| Teraspeed Modeling Services.
| http://www.teraspeed.com
[IBIS Ver]   4.0
[Comment Char] |_char
[File Name]   lpc15xxjbd100.ibs
[File Rev]   3.0
[Source]  Measured and created by Teraspeed Consulting Group LLC
[Date]   03-05-2014
[Notes]   Quality Check of this IBIS model: Model Passes IBIS Check
   Model parses into ICX IS. Simulation done with Hyperlynx.
   1. MIN TYP MAX information is based on Temperature and Voltage
   characteristics only.
   2. Package data measured using Tektronix IConnect Software.
[Disclaimer]
| Use: Teraspeed Consulting Group LLC ("Teraspeed") has
| licensed IBIS models to specific integrated circuit
| suppliers ("IC Vendors") for use and distribution as
| follows: Each IC Vendor may use IBIS Models, and distribute
| them to IC Vendor's customers to use solely for developing
| printed circuit board designs. Users of this model may
| modify the IBIS model to suit its specific applications but
| rights to derivative works and such modifications shall belong
| to Teraspeed. No other distribution of these materials is
| permitted.
| DISCLAIMER OF WARRANTY: UNLESS OTHERWISE AGREED TO IN WRITING
| TERASPEED DISCLAIMS AND USER WAIVES ALL WARRANTIES, EXPRESS
| OR IMPLIED, INCLUDING WARRANTIES OF MERCHANTABILITY AND
| FITNESS FOR A PARTICULAR PURPOSE. IN NO EVENT SHALL
| TERASPEED BE LIABLE FOR ANY DIRECT OR INDIRECT DAMAGES,
| WHETHER IN CONTRACT OR TORT, INCLUDING, WITHOUT LIMITATION,
| LOST PROFITS, BUSINESS INTERRUPTION, OR LOST INFORMATION
| ARISING OUT OF THE USE OF OR THE INABILITY TO USE THE MODEL,
| EVEN IF TERASPEED HAS BEEN ADVISED OF THE POSSIBILITY OF SUCH
| DAMAGES.
[Copyright]
| This file is the legal property of Teraspeed Copyright(c) 2014.
| All other rights are reserved.
[Component]LPC15xxJBD100
[Manufacturer] NXP Semiconductors
[Package]
| variable   typ   min   max
| qfp100
R_pkg  1.917E-02   1.414E-02   2.417E-02
L_pkg  3.087E-09   2.277E-09   3.891E-09
C_pkg  6.299E-13   4.647E-13   7.940E-13
[Pin] signal_name  model_name  R_pin  L_pin C_pin
1   PIO0_30 pio0_30 2.417E-02   3.891E-09   7.940E-13
2   PIO0_0  pio0_0  2.326E-02   3.745E-09   7.642E-13
3   PIO0_31 pio0_31 2.236E-02   3.600E-09   7.347E-13
4   VDD   POWER   2.147E-02   3.457E-09   7.055E-13
5   PIO1_0  pio1_0  2.059E-02   3.315E-09   6.766E-13
6   PIO0_1  pio0_1  1.972E-02   3.175E-09   6.480E-13
7   VSS   GND   1.887E-02   3.038E-09   6.200E-13
8   PIO0_2  pio0_2  1.803E-02   2.903E-09   5.923E-13
9   PIO1_12 pio1_12 1.721E-02   2.770E-09   5.653E-13
10   PIO0_3  pio0_3  1.640E-02   2.641E-09   5.389E-13
11   PIO1_13 pio1_13 1.562E-02   2.515E-09   5.132E-13
12   PIO1_14 pio1_14 1.487E-02   2.393E-09   4.885E-13
13   PIO0_4  pio0_4  1.414E-02   2.277E-09   4.647E-13
14   PIO0_5  pio0_5  1.487E-02   2.393E-09   4.885E-13
15   PIO1_15 pio1_15 1.562E-02   2.515E-09   5.132E-13
16   PIO0_6  pio0_6  1.640E-02   2.641E-09   5.389E-13
17   PIO0_7  pio0_7  1.721E-02   2.770E-09   5.653E-13
18   PIO1_16 pio1_16 1.803E-02   2.903E-09   5.923E-13
19   PIO0_8  pio0_8  1.887E-02   3.038E-09   6.200E-13
20   PIO1_17 pio1_17 1.972E-02   3.175E-09   6.480E-13
21   VREFP_ADC POWER 2.059E-02   3.315E-09   6.766E-13
22   VREFN   POWER   2.147E-02   3.457E-09   7.055E-13
23   PIO1_1  pio1_1  2.236E-02   3.600E-09   7.347E-13
24   PIO0_9  pio0_9  2.326E-02   3.745E-09   7.642E-13
25   PIO1_18 pio1_18 2.417E-02   3.891E-09   7.940E-13
26   PIO0_18 pio0_18 2.417E-02   3.891E-09   7.940E-13
27   VREFP_DAC_VDDCMP POWER  2.326E-02   3.745E-09   7.642E-13
28   PIO0_10 pio0_10 2.236E-02   3.600E-09   7.347E-13
29   PIO1_19 pio1_19 2.147E-02   3.457E-09   7.055E-13
30   VDDA   POWER   2.059E-02   3.315E-09   6.766E-13
31   VSSA   GND   1.972E-02   3.175E-09   6.480E-13
32   VDD   POWER   1.887E-02   3.038E-09   6.200E-13
33   PIO0_11 pio0_11 1.803E-02   2.903E-09   5.923E-13
34   PIO1_20 pio1_20 1.721E-02   2.770E-09   5.653E-13
35   PIO0_12 pio0_12 1.640E-02   2.641E-09   5.389E-13
36   PIO1_2  pio1_2  1.562E-02   2.515E-09   5.132E-13
37   PIO1_21 pio1_21 1.487E-02   2.393E-09   4.885E-13
38   PIO1_22 pio1_22 1.414E-02   2.277E-09   4.647E-13
39   VSS   GND   1.487E-02   2.393E-09   4.885E-13
40   VSS   GND   1.562E-02   2.515E-09   5.132E-13
41   PIO1_3  pio1_3  1.640E-02   2.641E-09   5.389E-13
42   PIO1_23 pio1_23 1.721E-02   2.770E-09   5.653E-13
43   PIO0_13 pio0_13 1.803E-02   2.903E-09   5.923E-13
44   PIO1_24 pio1_24 1.887E-02   3.038E-09   6.200E-13
45   PIO0_14 pio0_14 1.972E-02   3.175E-09   6.480E-13
46   PIO1_25 pio1_25 2.059E-02   3.315E-09   6.766E-13
47   PIO0_15 pio0_15 2.147E-02   3.457E-09   7.055E-13
48   PIO1_26 pio1_26 2.236E-02   3.600E-09   7.347E-13
49   PIO0_16 pio0_16 2.326E-02   3.745E-09   7.642E-13
50   PIO1_27 pio1_27 2.417E-02   3.891E-09   7.940E-13
51   PIO1_4  pio1_4  2.417E-02   3.891E-09   7.940E-13
52   PIO1_5  pio1_5  2.326E-02   3.745E-09   7.642E-13
53   XTALOUT term   2.236E-02   3.600E-09   7.347E-13
54   XTALIN  xtalin  2.147E-02   3.457E-09   7.055E-13
55   PIO1_28 pio1_28 2.059E-02   3.315E-09   6.766E-13
56   PIO1_29 pio1_29 1.972E-02   3.175E-09   6.480E-13
57   VDD   POWER   1.887E-02   3.038E-09   6.200E-13
58   PIO1_11 pio1_11 1.803E-02   2.903E-09   5.923E-13
59   PIO1_30 pio1_30 1.721E-02   2.770E-09   5.653E-13
60   PIO1_31 pio1_31 1.640E-02   2.641E-09   5.389E-13
61   PIO0_17 pio0_17 1.562E-02   2.515E-09   5.132E-13
62   PIO2_0  pio2_0  1.487E-02   2.393E-09   4.885E-13
63   PIO0_19 pio0_19 1.414E-02   2.277E-09   4.647E-13
64   PIO2_1  pio2_1  1.487E-02   2.393E-09   4.885E-13
65   VBAT   POWER   1.562E-02   2.515E-09   5.132E-13
66   RTCXIN  rtcxin  1.640E-02   2.641E-09   5.389E-13
67   RTCXOUT rtcxout 1.721E-02   2.770E-09   5.653E-13
68   VSS   GND   1.803E-02   2.903E-09   5.923E-13
69   PIO0_20 pio0_20 1.887E-02   3.038E-09   6.200E-13
70   VDD   POWER   1.972E-02   3.175E-09   6.480E-13
71   RESET   pio0_20 2.059E-02   3.315E-09   6.766E-13
72   PIO2_2  pio2_2  2.147E-02   3.457E-09   7.055E-13
73   PIO1_6  pio1_6  2.236E-02   3.600E-09   7.347E-13
74   PIO2_12 pio2_12 2.326E-02   3.745E-09   7.642E-13
75   PIO2_13 pio2_13 2.417E-02   3.891E-09   7.940E-13
76   PIO2_3  pio2_3  2.417E-02   3.891E-09   7.940E-13
77   PIO2_4  pio2_4  2.326E-02   3.745E-09   7.642E-13
78   PIO0_22 pio0_22 2.236E-02   3.600E-09   7.347E-13
79   PIO0_23 pio0_23 2.147E-02   3.457E-09   7.055E-13
80   PIO2_5  pio2_5  2.059E-02   3.315E-09   6.766E-13
81   PIO1_7  pio1_7  1.972E-02   3.175E-09   6.480E-13
82   PIO2_6  pio2_6  1.887E-02   3.038E-09   6.200E-13
83   VDD   POWER   1.803E-02   2.903E-09   5.923E-13
84   PIO1_8  pio1_8  1.721E-02   2.770E-09   5.653E-13
85   PIO1_9  pio1_9  1.640E-02   2.641E-09   5.389E-13
86   PIO2_7  pio2_7  1.562E-02   2.515E-09   5.132E-13
87   VSS   GND   1.487E-02   2.393E-09   4.885E-13
88   VSS   GND   1.414E-02   2.277E-09   4.647E-13
89   VDD   POWER   1.487E-02   2.393E-09   4.885E-13
90   PIO0_24 pio0_24 1.562E-02   2.515E-09   5.132E-13
91   PIO1_10 pio1_10 1.640E-02   2.641E-09   5.389E-13
92   PIO2_8  pio2_8  1.721E-02   2.770E-09   5.653E-13
93   PIO0_25 pio0_25 1.803E-02   2.903E-09   5.923E-13
94   PIO2_9  pio2_9  1.887E-02   3.038E-09   6.200E-13
95   PIO0_26 pio0_26 1.972E-02   3.175E-09   6.480E-13
96   PIO2_10 pio2_10 2.059E-02   3.315E-09   6.766E-13
97   PIO0_27 pio0_27 2.147E-02   3.457E-09   7.055E-13
98   PIO0_28 pio0_28 2.236E-02   3.600E-09   7.347E-13
99   PIO2_11 pio2_11 2.326E-02   3.745E-09   7.642E-13
100   PIO0_29 pio0_29 2.417E-02   3.891E-09   7.940E-13
[Model Selector]   pio0_0
pio_2.5v   GP io 2.5V
pio_3.3v   GP io 3.3V
pio_2.5v_pu   GP io 2.5V with pullup
pio_3.3v_pu   GP io 3.3V with pullup
pio_2.5v_pd   GP io 2.5V with pulldown
pio_3.3v_pd   GP io 3.3V with pulldown
[Model Selector]   pio0_1
pio_2.5v   GP io 2.5V
pio_3.3v   GP io 3.3V
pio_2.5v_pu   GP io 2.5V with pullup
pio_3.3v_pu   GP io 3.3V with pullup
pio_2.5v_pd   GP io 2.5V with pulldown
pio_3.3v_pd   GP io 3.3V with pulldown
[Model Selector]   pio0_2
pio_2.5v   GP io 2.5V
pio_3.3v   GP io 3.3V
pio_2.5v_pu   GP io 2.5V with pullup
pio_3.3v_pu   GP io 3.3V with pullup
pio_2.5v_pd   GP io 2.5V with pulldown
pio_3.3v_pd   GP io 3.3V with pulldown
[Model Selector]   pio0_3
pio_2.5v   GP io 2.5V
pio_3.3v   GP io 3.3V
pio_2.5v_pu   GP io 2.5V with pullup
pio_3.3v_pu   GP io 3.3V with pullup
pio_2.5v_pd   GP io 2.5V with pulldown
pio_3.3v_pd   GP io 3.3V with pulldown
[Model Selector]   pio0_4
pio_2.5v   GP io 2.5V
pio_3.3v   GP io 3.3V
pio_2.5v_pu   GP io 2.5V with pullup
pio_3.3v_pu   GP io 3.3V with pullup
pio_2.5v_pd   GP io 2.5V with pulldown
pio_3.3v_pd   GP io 3.3V with pulldown
[Model Selector]   pio0_5
pio_2.5v   GP io 2.5V
pio_3.3v   GP io 3.3V
pio_2.5v_pu   GP io 2.5V with pullup
pio_3.3v_pu   GP io 3.3V with pullup
pio_2.5v_pd   GP io 2.5V with pulldown
pio_3.3v_pd   GP io 3.3V with pulldown
[Model Selector]   pio0_6
pio_2.5v   GP io 2.5V
pio_3.3v   GP io 3.3V
pio_2.5v_pu   GP io 2.5V with pullup
pio_3.3v_pu   GP io 3.3V with pullup
pio_2.5v_pd   GP io 2.5V with pulldown
pio_3.3v_pd   GP io 3.3V with pulldown
[Model Selector]   pio0_7
pio_2.5v   GP io 2.5V
pio_3.3v   GP io 3.3V
pio_2.5v_pu   GP io 2.5V with pullup
pio_3.3v_pu   GP io 3.3V with pullup
pio_2.5v_pd   GP io 2.5V with pulldown
pio_3.3v_pd   GP io 3.3V with pulldown
[Model Selector]   pio0_8
pio_2.5v   GP io 2.5V
pio_3.3v   GP io 3.3V
pio_2.5v_pu   GP io 2.5V with pullup
pio_3.3v_pu   GP io 3.3V with pullup
pio_2.5v_pd   GP io 2.5V with pulldown
pio_3.3v_pd   GP io 3.3V with pulldown
[Model Selector]   pio0_9
pio_2.5v   GP io 2.5V
pio_3.3v   GP io 3.3V
pio_2.5v_pu   GP io 2.5V with pullup
pio_3.3v_pu   GP io 3.3V with pullup
pio_2.5v_pd   GP io 2.5V with pulldown
pio_3.3v_pd   GP io 3.3V with pulldown
[Model Selector]   pio0_10
pio_2.5v   GP io 2.5V
pio_3.3v   GP io 3.3V
pio_2.5v_pu   GP io 2.5V with pullup
pio_3.3v_pu   GP io 3.3V with pullup
pio_2.5v_pd   GP io 2.5V with pulldown
pio_3.3v_pd   GP io 3.3V with pulldown
[Model Selector]   pio0_11
pio_2.5v   GP io 2.5V
pio_3.3v   GP io 3.3V
pio_2.5v_pu   GP io 2.5V with pullup
pio_3.3v_pu   GP io 3.3V with pullup
pio_2.5v_pd   GP io 2.5V with pulldown
pio_3.3v_pd   GP io 3.3V with pulldown
[Model Selector]   pio0_12
pio_2.5v   GP io 2.5V
pio_3.3v   GP io 3.3V
pio_2.5v_pu   GP io 2.5V with pullup
pio_3.3v_pu   GP io 3.3V with pullup
pio_2.5v_pd   GP io 2.5V with pulldown
pio_3.3v_pd   GP io 3.3V with pulldown
[Model Selector]   pio0_13
pio_2.5v   GP io 2.5V
pio_3.3v   GP io 3.3V
pio_2.5v_pu   GP io 2.5V with pullup
pio_3.3v_pu   GP io 3.3V with pullup
pio_2.5v_pd   GP io 2.5V with pulldown
pio_3.3v_pd   GP io 3.3V with pulldown
[Model Selector]   pio0_14
pio_2.5v   GP io 2.5V
pio_3.3v   GP io 3.3V
pio_2.5v_pu   GP io 2.5V with pullup
pio_3.3v_pu   GP io 3.3V with pullup
pio_2.5v_pd   GP io 2.5V with pulldown
pio_3.3v_pd   GP io 3.3V with pulldown
[Model Selector]   pio0_15
pio_2.5v   GP io 2.5V
pio_3.3v   GP io 3.3V
pio_2.5v_pu   GP io 2.5V with pullup
pio_3.3v_pu   GP io 3.3V with pullup
pio_2.5v_pd   GP io 2.5V with pulldown
pio_3.3v_pd   GP io 3.3V with pulldown
[Model Selector]   pio0_16
pio_2.5v   GP io 2.5V
pio_3.3v   GP io 3.3V
pio_2.5v_pu   GP io 2.5V with pullup
pio_3.3v_pu   GP io 3.3V with pullup
pio_2.5v_pd   GP io 2.5V with pulldown
pio_3.3v_pd   GP io 3.3V with pulldown
[Model Selector]   pio0_17
pio_2.5v   GP io 2.5V
pio_3.3v   GP io 3.3V
pio_2.5v_pu   GP io 2.5V with pullup
pio_3.3v_pu   GP io 3.3V with pullup
pio_2.5v_pd   GP io 2.5V with pulldown
pio_3.3v_pd   GP io 3.3V with pulldown
[Model Selector]   pio0_18
pio_2.5v   GP io 2.5V
pio_3.3v   GP io 3.3V
pio_2.5v_pu   GP io 2.5V with pullup
pio_3.3v_pu   GP io 3.3V with pullup
pio_2.5v_pd   GP io 2.5V with pulldown
pio_3.3v_pd   GP io 3.3V with pulldown
[Model Selector]   pio0_19
pio_2.5v   GP io 2.5V
pio_3.3v   GP io 3.3V
pio_2.5v_pu   GP io 2.5V with pullup
pio_3.3v_pu   GP io 3.3V with pullup
pio_2.5v_pd   GP io 2.5V with pulldown
pio_3.3v_pd   GP io 3.3V with pulldown
[Model Selector]   pio0_20
pio_2.5v   GP io 2.5V
pio_3.3v   GP io 3.3V
pio_2.5v_pu   GP io 2.5V with pullup
pio_3.3v_pu   GP io 3.3V with pullup
pio_2.5v_pd   GP io 2.5V with pulldown
pio_3.3v_pd   GP io 3.3V with pulldown
[Model Selector]   pio0_21
pio_2.5v   GP io 2.5V
pio_3.3v   GP io 3.3V
pio_2.5v_pu   GP io 2.5V with pullup
pio_3.3v_pu   GP io 3.3V with pullup
pio_2.5v_pd   GP io 2.5V with pulldown
pio_3.3v_pd   GP io 3.3V with pulldown
resetb_in_2.5v  2.5V reset input
resetb_in_3.3v  3.3V reset input
[Model Selector]   pio0_22
pio_2.5v   GP io 2.5V
pio_3.3v   GP io 3.3V
pio_2.5v_pu   GP io 2.5V with pullup
pio_3.3v_pu   GP io 3.3V with pullup
pio_2.5v_pd   GP io 2.5V with pulldown
pio_3.3v_pd   GP io 3.3V with pulldown
i2c_std_fst_2.5v   I2C Open Drain io 2.5V
i2c_std_fst_3.3v   I2C Open Drain io 3.3V
[Model Selector]   pio0_23
pio_2.5v   GP io 2.5V
pio_3.3v   GP io 3.3V
pio_2.5v_pu   GP io 2.5V with pullup
pio_3.3v_pu   GP io 3.3V with pullup
pio_2.5v_pd   GP io 2.5V with pulldown
pio_3.3v_pd   GP io 3.3V with pulldown
i2c_std_fst_2.5v   I2C Open Drain io 2.5V
i2c_std_fst_3.3v   I2C Open Drain io 3.3V
[Model Selector]   pio0_24
hd_pio_2.5v   High Drive GP io 2.5V
hd_pio_3.3v   High Drive GP io 3.3V
hd_pio_2.5v_pu  High Drive GP io 2.5V with pullup
hd_pio_3.3v_pu  High Drive GP io 3.3V with pullup
hd_pio_2.5v_pd  High Drive GP io 2.5V with pulldown
hd_pio_3.3v_pd  High Drive GP io 3.3V with pulldown
[Model Selector]   pio0_25
pio_2.5v   GP io 2.5V
pio_3.3v   GP io 3.3V
pio_2.5v_pu   GP io 2.5V with pullup
pio_3.3v_pu   GP io 3.3V with pullup
pio_2.5v_pd   GP io 2.5V with pulldown
pio_3.3v_pd   GP io 3.3V with pulldown
[Model Selector]   pio0_26
pio_2.5v   GP io 2.5V
pio_3.3v   GP io 3.3V
pio_2.5v_pu   GP io 2.5V with pullup
pio_3.3v_pu   GP io 3.3V with pullup
pio_2.5v_pd   GP io 2.5V with pulldown
pio_3.3v_pd   GP io 3.3V with pulldown
[Model Selector]   pio0_27
pio_2.5v   GP io 2.5V
pio_3.3v   GP io 3.3V
pio_2.5v_pu   GP io 2.5V with pullup
pio_3.3v_pu   GP io 3.3V with pullup
pio_2.5v_pd   GP io 2.5V with pulldown
pio_3.3v_pd   GP io 3.3V with pulldown
[Model Selector]   pio0_28
pio_2.5v   GP io 2.5V
pio_3.3v   GP io 3.3V
pio_2.5v_pu   GP io 2.5V with pullup
pio_3.3v_pu   GP io 3.3V with pullup
pio_2.5v_pd   GP io 2.5V with pulldown
pio_3.3v_pd   GP io 3.3V with pulldown
[Model Selector]   pio0_29
pio_2.5v   GP io 2.5V
pio_3.3v   GP io 3.3V
pio_2.5v_pu   GP io 2.5V with pullup
pio_3.3v_pu   GP io 3.3V with pullup
pio_2.5v_pd   GP io 2.5V with pulldown
pio_3.3v_pd   GP io 3.3V with pulldown
[Model Selector]   pio0_30
pio_2.5v   GP io 2.5V
pio_3.3v   GP io 3.3V
pio_2.5v_pu   GP io 2.5V with pullup
pio_3.3v_pu   GP io 3.3V with pullup
pio_2.5v_pd   GP io 2.5V with pulldown
pio_3.3v_pd   GP io 3.3V with pulldown
[Model Selector]   pio0_31
pio_2.5v   GP io 2.5V
pio_3.3v   GP io 3.3V
pio_2.5v_pu   GP io 2.5V with pullup
pio_3.3v_pu   GP io 3.3V with pullup
pio_2.5v_pd   GP io 2.5V with pulldown
pio_3.3v_pd   GP io 3.3V with pulldown
[Model Selector]   pio1_0
pio_2.5v   GP io 2.5V
pio_3.3v   GP io 3.3V
pio_2.5v_pu   GP io 2.5V with pullup
pio_3.3v_pu   GP io 3.3V with pullup
pio_2.5v_pd   GP io 2.5V with pulldown
pio_3.3v_pd   GP io 3.3V with pulldown
[Model Selector]   pio1_1
pio_2.5v   GP io 2.5V
pio_3.3v   GP io 3.3V
pio_2.5v_pu   GP io 2.5V with pullup
pio_3.3v_pu   GP io 3.3V with pullup
pio_2.5v_pd   GP io 2.5V with pulldown
pio_3.3v_pd   GP io 3.3V with pulldown
[Model Selector]   pio1_2
pio_2.5v   GP io 2.5V
pio_3.3v   GP io 3.3V
pio_2.5v_pu   GP io 2.5V with pullup
pio_3.3v_pu   GP io 3.3V with pullup
pio_2.5v_pd   GP io 2.5V with pulldown
pio_3.3v_pd   GP io 3.3V with pulldown
[Model Selector]   pio1_3
pio_2.5v   GP io 2.5V
pio_3.3v   GP io 3.3V
pio_2.5v_pu   GP io 2.5V with pullup
pio_3.3v_pu   GP io 3.3V with pullup
pio_2.5v_pd   GP io 2.5V with pulldown
pio_3.3v_pd   GP io 3.3V with pulldown
[Model Selector]   pio1_4
pio_2.5v   GP io 2.5V
pio_3.3v   GP io 3.3V
pio_2.5v_pu   GP io 2.5V with pullup
pio_3.3v_pu   GP io 3.3V with pullup
pio_2.5v_pd   GP io 2.5V with pulldown
pio_3.3v_pd   GP io 3.3V with pulldown
[Model Selector]   pio1_5
pio_2.5v   GP io 2.5V
pio_3.3v   GP io 3.3V
pio_2.5v_pu   GP io 2.5V with pullup
pio_3.3v_pu   GP io 3.3V with pullup
pio_2.5v_pd   GP io 2.5V with pulldown
pio_3.3v_pd   GP io 3.3V with pulldown
[Model Selector]   pio1_6
pio_2.5v   GP io 2.5V
pio_3.3v   GP io 3.3V
pio_2.5v_pu   GP io 2.5V with pullup
pio_3.3v_pu   GP io 3.3V with pullup
pio_2.5v_pd   GP io 2.5V with pulldown
pio_3.3v_pd   GP io 3.3V with pulldown
[Model Selector]   pio1_7
pio_2.5v   GP io 2.5V
pio_3.3v   GP io 3.3V
pio_2.5v_pu   GP io 2.5V with pullup
pio_3.3v_pu   GP io 3.3V with pullup
pio_2.5v_pd   GP io 2.5V with pulldown
pio_3.3v_pd   GP io 3.3V with pulldown
[Model Selector]   pio1_8
pio_2.5v   GP io 2.5V
pio_3.3v   GP io 3.3V
pio_2.5v_pu   GP io 2.5V with pullup
pio_3.3v_pu   GP io 3.3V with pullup
pio_2.5v_pd   GP io 2.5V with pulldown
pio_3.3v_pd   GP io 3.3V with pulldown
[Model Selector]   pio1_9
pio_2.5v   GP io 2.5V
pio_3.3v   GP io 3.3V
pio_2.5v_pu   GP io 2.5V with pullup
pio_3.3v_pu   GP io 3.3V with pullup
pio_2.5v_pd   GP io 2.5V with pulldown
pio_3.3v_pd   GP io 3.3V with pulldown
[Model Selector]   pio1_10
pio_2.5v   GP io 2.5V
pio_3.3v   GP io 3.3V
pio_2.5v_pu   GP io 2.5V with pullup
pio_3.3v_pu   GP io 3.3V with pullup
pio_2.5v_pd   GP io 2.5V with pulldown
pio_3.3v_pd   GP io 3.3V with pulldown
[Model Selector]   pio1_11
pio_2.5v   GP io 2.5V
pio_3.3v   GP io 3.3V
pio_2.5v_pu   GP io 2.5V with pullup
pio_3.3v_pu   GP io 3.3V with pullup
pio_2.5v_pd   GP io 2.5V with pulldown
pio_3.3v_pd   GP io 3.3V with pulldown
[Model Selector]   pio1_12
pio_2.5v   GP io 2.5V
pio_3.3v   GP io 3.3V
pio_2.5v_pu   GP io 2.5V with pullup
pio_3.3v_pu   GP io 3.3V with pullup
pio_2.5v_pd   GP io 2.5V with pulldown
pio_3.3v_pd   GP io 3.3V with pulldown
[Model Selector]   pio1_13
pio_2.5v   GP io 2.5V
pio_3.3v   GP io 3.3V
pio_2.5v_pu   GP io 2.5V with pullup
pio_3.3v_pu   GP io 3.3V with pullup
pio_2.5v_pd   GP io 2.5V with pulldown
pio_3.3v_pd   GP io 3.3V with pulldown
[Model Selector]   pio1_14
pio_2.5v   GP io 2.5V
pio_3.3v   GP io 3.3V
pio_2.5v_pu   GP io 2.5V with pullup
pio_3.3v_pu   GP io 3.3V with pullup
pio_2.5v_pd   GP io 2.5V with pulldown
pio_3.3v_pd   GP io 3.3V with pulldown
[Model Selector]   pio1_15
pio_2.5v   GP io 2.5V
pio_3.3v   GP io 3.3V
pio_2.5v_pu   GP io 2.5V with pullup
pio_3.3v_pu   GP io 3.3V with pullup
pio_2.5v_pd   GP io 2.5V with pulldown
pio_3.3v_pd   GP io 3.3V with pulldown
[Model Selector]   pio1_16
pio_2.5v   GP io 2.5V
pio_3.3v   GP io 3.3V
pio_2.5v_pu   GP io 2.5V with pullup
pio_3.3v_pu   GP io 3.3V with pullup
pio_2.5v_pd   GP io 2.5V with pulldown
pio_3.3v_pd   GP io 3.3V with pulldown
[Model Selector]   pio1_17
pio_2.5v   GP io 2.5V
pio_3.3v   GP io 3.3V
pio_2.5v_pu   GP io 2.5V with pullup
pio_3.3v_pu   GP io 3.3V with pullup
pio_2.5v_pd   GP io 2.5V with pulldown
pio_3.3v_pd   GP io 3.3V with pulldown
[Model Selector]   pio1_18
pio_2.5v   GP io 2.5V
pio_3.3v   GP io 3.3V
pio_2.5v_pu   GP io 2.5V with pullup
pio_3.3v_pu   GP io 3.3V with pullup
pio_2.5v_pd   GP io 2.5V with pulldown
pio_3.3v_pd   GP io 3.3V with pulldown
[Model Selector]   pio1_19
pio_2.5v   GP io 2.5V
pio_3.3v   GP io 3.3V
pio_2.5v_pu   GP io 2.5V with pullup
pio_3.3v_pu   GP io 3.3V with pullup
pio_2.5v_pd   GP io 2.5V with pulldown
pio_3.3v_pd   GP io 3.3V with pulldown
[Model Selector]   pio1_20
pio_2.5v   GP io 2.5V
pio_3.3v   GP io 3.3V
pio_2.5v_pu   GP io 2.5V with pullup
pio_3.3v_pu   GP io 3.3V with pullup
pio_2.5v_pd   GP io 2.5V with pulldown
pio_3.3v_pd   GP io 3.3V with pulldown
[Model Selector]   pio1_21
pio_2.5v   GP io 2.5V
pio_3.3v   GP io 3.3V
pio_2.5v_pu   GP io 2.5V with pullup
pio_3.3v_pu   GP io 3.3V with pullup
pio_2.5v_pd   GP io 2.5V with pulldown
pio_3.3v_pd   GP io 3.3V with pulldown
[Model Selector]   pio1_22
pio_2.5v   GP io 2.5V
pio_3.3v   GP io 3.3V
pio_2.5v_pu   GP io 2.5V with pullup
pio_3.3v_pu   GP io 3.3V with pullup
pio_2.5v_pd   GP io 2.5V with pulldown
pio_3.3v_pd   GP io 3.3V with pulldown
[Model Selector]   pio1_23
pio_2.5v   GP io 2.5V
pio_3.3v   GP io 3.3V
pio_2.5v_pu   GP io 2.5V with pullup
pio_3.3v_pu   GP io 3.3V with pullup
pio_2.5v_pd   GP io 2.5V with pulldown
pio_3.3v_pd   GP io 3.3V with pulldown
[Model Selector]   pio1_24
pio_2.5v   GP io 2.5V
pio_3.3v   GP io 3.3V
pio_2.5v_pu   GP io 2.5V with pullup
pio_3.3v_pu   GP io 3.3V with pullup
pio_2.5v_pd   GP io 2.5V with pulldown
pio_3.3v_pd   GP io 3.3V with pulldown
[Model Selector]   pio1_25
pio_2.5v   GP io 2.5V
pio_3.3v   GP io 3.3V
pio_2.5v_pu   GP io 2.5V with pullup
pio_3.3v_pu   GP io 3.3V with pullup
pio_2.5v_pd   GP io 2.5V with pulldown
pio_3.3v_pd   GP io 3.3V with pulldown
[Model Selector]   pio1_26
pio_2.5v   GP io 2.5V
pio_3.3v   GP io 3.3V
pio_2.5v_pu   GP io 2.5V with pullup
pio_3.3v_pu   GP io 3.3V with pullup
pio_2.5v_pd   GP io 2.5V with pulldown
pio_3.3v_pd   GP io 3.3V with pulldown
[Model Selector]   pio1_27
pio_2.5v   GP io 2.5V
pio_3.3v   GP io 3.3V
pio_2.5v_pu   GP io 2.5V with pullup
pio_3.3v_pu   GP io 3.3V with pullup
pio_2.5v_pd   GP io 2.5V with pulldown
pio_3.3v_pd   GP io 3.3V with pulldown
[Model Selector]   pio1_28
pio_2.5v   GP io 2.5V
pio_3.3v   GP io 3.3V
pio_2.5v_pu   GP io 2.5V with pullup
pio_3.3v_pu   GP io 3.3V with pullup
pio_2.5v_pd   GP io 2.5V with pulldown
pio_3.3v_pd   GP io 3.3V with pulldown
[Model Selector]   pio1_29
pio_2.5v   GP io 2.5V
pio_3.3v   GP io 3.3V
pio_2.5v_pu   GP io 2.5V with pullup
pio_3.3v_pu   GP io 3.3V with pullup
pio_2.5v_pd   GP io 2.5V with pulldown
pio_3.3v_pd   GP io 3.3V with pulldown
[Model Selector]   pio1_30
pio_2.5v   GP io 2.5V
pio_3.3v   GP io 3.3V
pio_2.5v_pu   GP io 2.5V with pullup
pio_3.3v_pu   GP io 3.3V with pullup
pio_2.5v_pd   GP io 2.5V with pulldown
pio_3.3v_pd   GP io 3.3V with pulldown
[Model Selector]   pio1_31
pio_2.5v   GP io 2.5V
pio_3.3v   GP io 3.3V
pio_2.5v_pu   GP io 2.5V with pullup
pio_3.3v_pu   GP io 3.3V with pullup
pio_2.5v_pd   GP io 2.5V with pulldown
pio_3.3v_pd   GP io 3.3V with pulldown
[Model Selector]   pio2_0
pio_2.5v   GP io 2.5V
pio_3.3v   GP io 3.3V
pio_2.5v_pu   GP io 2.5V with pullup
pio_3.3v_pu   GP io 3.3V with pullup
pio_2.5v_pd   GP io 2.5V with pulldown
pio_3.3v_pd   GP io 3.3V with pulldown
[Model Selector]   pio2_1
pio_2.5v   GP io 2.5V
pio_3.3v   GP io 3.3V
pio_2.5v_pu   GP io 2.5V with pullup
pio_3.3v_pu   GP io 3.3V with pullup
pio_2.5v_pd   GP io 2.5V with pulldown
pio_3.3v_pd   GP io 3.3V with pulldown
[Model Selector]   pio2_2
pio_2.5v   GP io 2.5V
pio_3.3v   GP io 3.3V
pio_2.5v_pu   GP io 2.5V with pullup
pio_3.3v_pu   GP io 3.3V with pullup
pio_2.5v_pd   GP io 2.5V with pulldown
pio_3.3v_pd   GP io 3.3V with pulldown
[Model Selector]   pio2_3
pio_2.5v   GP io 2.5V
pio_3.3v   GP io 3.3V
pio_2.5v_pu   GP io 2.5V with pullup
pio_3.3v_pu   GP io 3.3V with pullup
pio_2.5v_pd   GP io 2.5V with pulldown
pio_3.3v_pd   GP io 3.3V with pulldown
[Model Selector]   pio2_4
pio_2.5v   GP io 2.5V
pio_3.3v   GP io 3.3V
pio_2.5v_pu   GP io 2.5V with pullup
pio_3.3v_pu   GP io 3.3V with pullup
pio_2.5v_pd   GP io 2.5V with pulldown
pio_3.3v_pd   GP io 3.3V with pulldown
[Model Selector]   pio2_5
pio_2.5v   GP io 2.5V
pio_3.3v   GP io 3.3V
pio_2.5v_pu   GP io 2.5V with pullup
pio_3.3v_pu   GP io 3.3V with pullup
pio_2.5v_pd   GP io 2.5V with pulldown
pio_3.3v_pd   GP io 3.3V with pulldown
[Model Selector]   pio2_6
pio_2.5v   GP io 2.5V
pio_3.3v   GP io 3.3V
pio_2.5v_pu   GP io 2.5V with pullup
pio_3.3v_pu   GP io 3.3V with pullup
pio_2.5v_pd   GP io 2.5V with pulldown
pio_3.3v_pd   GP io 3.3V with pulldown
[Model Selector]   pio2_7
pio_2.5v   GP io 2.5V
pio_3.3v   GP io 3.3V
pio_2.5v_pu   GP io 2.5V with pullup
pio_3.3v_pu   GP io 3.3V with pullup
pio_2.5v_pd   GP io 2.5V with pulldown
pio_3.3v_pd   GP io 3.3V with pulldown
[Model Selector]   pio2_8
pio_2.5v   GP io 2.5V
pio_3.3v   GP io 3.3V
pio_2.5v_pu   GP io 2.5V with pullup
pio_3.3v_pu   GP io 3.3V with pullup
pio_2.5v_pd   GP io 2.5V with pulldown
pio_3.3v_pd   GP io 3.3V with pulldown
[Model Selector]   pio2_9
pio_2.5v   GP io 2.5V
pio_3.3v   GP io 3.3V
pio_2.5v_pu   GP io 2.5V with pullup
pio_3.3v_pu   GP io 3.3V with pullup
pio_2.5v_pd   GP io 2.5V with pulldown
pio_3.3v_pd   GP io 3.3V with pulldown
[Model Selector]   pio2_10
pio_2.5v   GP io 2.5V
pio_3.3v   GP io 3.3V
pio_2.5v_pu   GP io 2.5V with pullup
pio_3.3v_pu   GP io 3.3V with pullup
pio_2.5v_pd   GP io 2.5V with pulldown
pio_3.3v_pd   GP io 3.3V with pulldown
[Model Selector]   pio2_11
pio_2.5v   GP io 2.5V
pio_3.3v   GP io 3.3V
pio_2.5v_pu   GP io 2.5V with pullup
pio_3.3v_pu   GP io 3.3V with pullup
pio_2.5v_pd   GP io 2.5V with pulldown
pio_3.3v_pd   GP io 3.3V with pulldown
[Model Selector]   pio2_12
pio_2.5v   GP io 2.5V
pio_3.3v   GP io 3.3V
pio_2.5v_pu   GP io 2.5V with pullup
pio_3.3v_pu   GP io 3.3V with pullup
pio_2.5v_pd   GP io 2.5V with pulldown
pio_3.3v_pd   GP io 3.3V with pulldown
[Model Selector]   pio2_13
pio_2.5v   GP io 2.5V
pio_3.3v   GP io 3.3V
pio_2.5v_pu   GP io 2.5V with pullup
pio_3.3v_pu   GP io 3.3V with pullup
pio_2.5v_pd   GP io 2.5V with pulldown
pio_3.3v_pd   GP io 3.3V with pulldown
[Model Selector]   rtcxin
rtcx_2.5v   Real Time Clock 2.5V input
rtcx_3.3v   Real Time Clock 3.3V input
[Model Selector]   rtcxout
out_2.5v   Real Time Clock 2.5V output
out_3.3v   Real Time Clock 3.3V output
[Model Selector]   usb
usb1_np_2.5v   usb1 io,np,2.5v
usb1_np_3.3v   usb1 io,np,3.3v
usb1_pd_2.5v   usb1 io,pd,2.5v
usb1_pd_3.3v   usb1 io,pd,3.3v
[Model Selector] xtalin
xtal_2.5v   2.5V crystal osc input
xtal_3.3v   3.3V crystal osc input
[Model] term
Model_type Terminator
C_comp  0pF 0pF 0pF
| variable typ   min   max
[Voltage Range]   3.30000V  3.00000V  3.60000V
[POWER Clamp Reference]  3.30000V  3.00000V  3.60000V
[GND Clamp Reference]   0.00000V  0.00000V  0.00000V
[Temperature Range]   25   85   -40
| Models and submodels in the file (27): hd_pio_2.5v (Input), hd_pio_2.5v_pd (Input), hd_pio_2.5v_pu (Input), hd_pio_3.3v (Input), hd_pio_3.3v_pd (Input), hd_pio_3.3v_pu (Input), pio_2.5v (Input), pio_2.5v_pd (Input), pio_2.5v_pu (Input), pio_3.3v (Input), pio_3.3v_pd (Input), pio_3.3v_pu (Input), resetb_in_2.5v (Input), resetb_in_3.3v (Input), rtcx_2.5v (Input), rtcx_3.3v (Input), xtal_2.5v (Input), xtal_3.3v (Input), i2c_std_fst_2.5v (I/O_open_drain), i2c_std_fst_3.3v (I/O_open_drain), usb1_np_2.5v (I/O), usb1_pd_2.5v (I/O), usb1_np_3.3v (I/O), usb1_pd_3.3v (I/O), out_2.5v (I/O), out_3.3v (I/O), term (Terminator)
